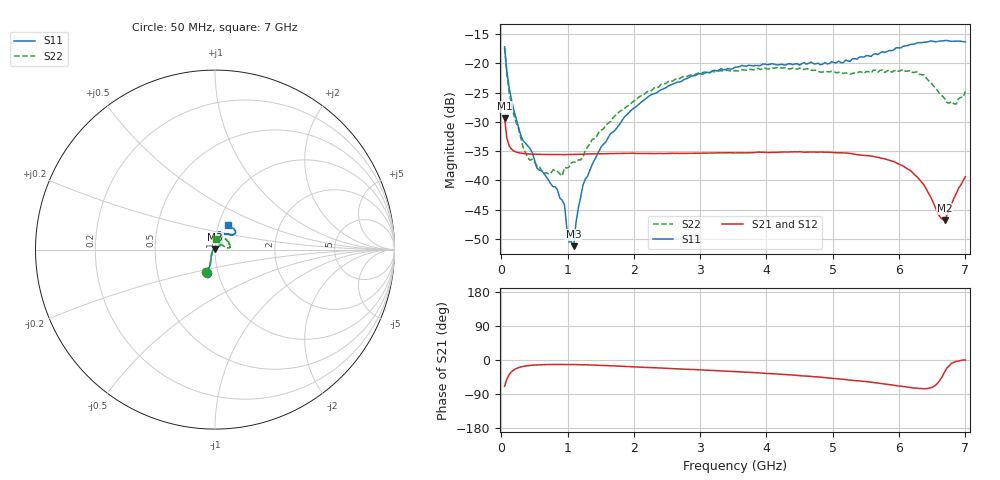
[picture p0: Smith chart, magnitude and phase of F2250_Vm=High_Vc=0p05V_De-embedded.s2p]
! Integrated Device Technology
! Corporate Headquarters
! 6024 Silver Creek Valley Road
! San Jose, CA 95138  USA
! Phone:  1-408-284-8200
! Toll Free:  1-800-223-1366
! Webpage:  http://www.idt.com/
! Timing and RF Division
! 515 Groton Road, Suite 102
! Westford, MA 01886-6024
! Device:  F2250
! Description: Voltage Variable RF Attenuator
! Frequency:  50.0 -  6000.00 MHz
! Package:  3x3 mm Thin QFN Plastic Package: 16 pin
! Ports:  2 RF, 3 DC
!  Pin  1  = GND
!  Pin  2  = NC
!  Pin  3  = RF1  = Port 1
!  Pin  4  = NC
!  Pin  5  = GND
!  Pin  6  = GND
!  Pin  7  = GND
!  Pin  8  = GND
!  Pin  9  = NC
!  Pin 10  = RF2  = Port 2
!  Pin 11  = NC
!  Pin 12  = GND
!  Pin 13  = GND
!  Pin 14  = VCNTRL
!  Pin 15  = VDD
!  Pin 16  = VMODE
! Vcntrl:  0.050 Volts
! Vmode:  +3.300 Volts
! Vdd:  +3.30  Volts
! Current:  1.243 mA
! Data:  The device was measured on a the F2250 evaluation board which has
!  individual transmission lines to the RF pins.  Data was collected
!  using a calibrated network analyzer.  The evaluation board was
!  de-embedded using a TRL calibration technique.
!  The reference plane is the edge of the package pin.
! Misc:  SN 10
!  Action Tracker AT0258
! Date Measured:  2014-11-26
! Date:  2015-10-15  MJV
! Note:
!  Integrated Device Technology supplies this data as a sample of measured
!  data at the package pin for this product.  Your particular data for this
!  product may vary.
!  Data was taken at 25 degrees C.
!  Integrated Device Technology reserves the right to change this data at anytime.
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# GHz S dB R 50
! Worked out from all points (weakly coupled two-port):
!   201 points, 50 MHz to 7 GHz, reference 50 ohm
!   highest |S21| = -29.38 dB at 50 MHz (marker M1); lowest = -46.8 dB at 6.687 GHz (marker M2)
!   lowest |S11| = -51.2 dB at 1.093 GHz (marker M3), VSWR 1.01, Z = 50 + j0.274 ohm
!   |S11| at or under -10 dB: start of sweep to end of sweep
!   |S22| runs from -39.2 to -17.4 dB; largest |S21 - S12| = 6.1e-05
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0.05  -17.18 -108.5  -29.38 -69.5  -29.38 -69.5  -17.37 -110.6
0.08475  -21.47 -107.4  -32.86 -50.1  -32.86 -50.1  -21.87 -109.0
0.15425  -26.23 -116.6  -34.68 -31.0  -34.68 -31.0  -27.10 -120.7
0.29325  -32.28 -127.4  -35.35 -18.5  -35.35 -18.4  -32.67 -133.5
0.3975  -34.11 -142.2  -35.48 -15.0  -35.48 -15.1  -36.08 -158.3
0.5365  -37.87 -154.6  -35.55 -12.9  -35.55 -12.9  -37.49 -180.0
0.64075  -38.78 -162.6  -35.58 -12.2  -35.58 -12.2  -38.86 160.6
0.91875  -43.38 155.9  -35.60 -11.8  -35.60 -11.8  -39.22 127.9
0.9535  -44.23 170.8  -35.60 -11.8  -35.60 -11.8  -37.81 124.1
1.023  -50.54 140.8  -35.59 -11.9  -35.59 -11.9  -37.72 108.0
1.0925  -51.25 88.6  -35.57 -12.0  -35.57 -12.0  -36.85 98.8
1.12725  -47.17 61.8  -35.56 -12.1  -35.56 -12.1  -36.93 91.6
1.2315  -40.84 40.9  -35.52 -12.5  -35.52 -12.5  -36.05 77.4
1.6485  -32.02 41.3  -35.43 -15.2  -35.44 -15.2  -29.92 60.0
2.37825  -24.75 46.7  -35.39 -21.0  -35.40 -21.1  -24.03 53.9
3.525  -20.66 71.7  -35.32 -30.6  -35.32 -30.6  -21.26 72.9
4.7065  -20.06 72.0  -35.16 -43.9  -35.16 -43.9  -21.20 70.4
5.85325  -17.79 40.5  -36.58 -64.8  -36.58 -64.9  -21.13 23.4
6.27025  -16.53 39.4  -39.39 -74.5  -39.40 -74.6  -21.46 8.6
6.68725  -16.11 47.9  -46.80 -31.1  -46.78 -30.8  -26.03 28.4
6.861  -16.21 54.5  -42.30 -3.7  -42.27 -3.7  -26.96 57.4
7  -16.32 62.4  -39.36 -0.1  -39.32 -0.3  -24.82 83.6
